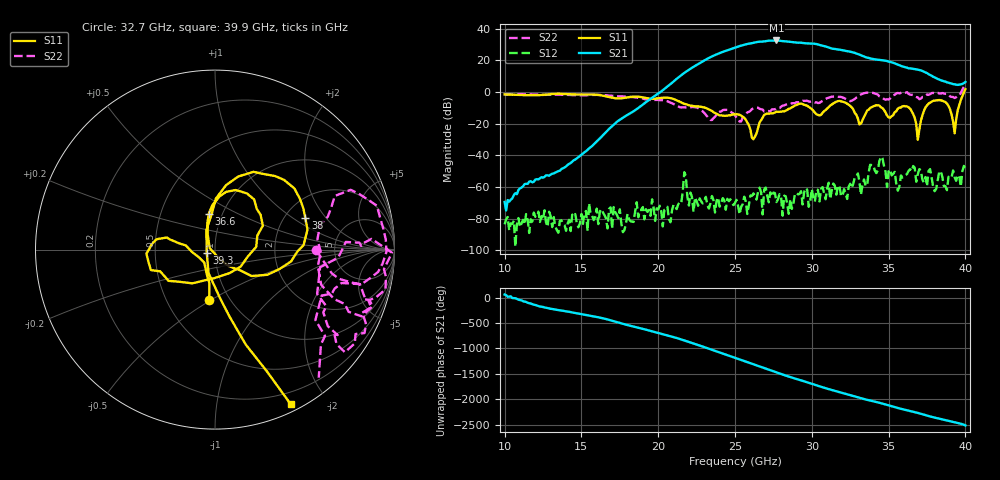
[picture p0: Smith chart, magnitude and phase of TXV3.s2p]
!Keysight Technologies,M9808A,MY58100618,A.14.70.03
!Date: Monday, February 27, 2023 13:37:35
!Correction: S11(C  2-Port  )
!S21(C  2-Port  )
!S12(C  2-Port  )
!S22(C  2-Port  )
!S2P File: Measurements: S11, S21, S12, S22:
# Hz S  RI  R 50
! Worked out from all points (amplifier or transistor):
!   301 points, 10 GHz to 40 GHz, reference 50 ohm
!   highest |S21| = 32.6 dB at 27.7 GHz (marker M1)
!   |S21| within 3 dB of that: 25.49 GHz to 30.57 GHz (5.074 GHz wide, 18.1 % of centre)
!   unconditionally stable (mu >= 1): start of sweep to 33.74 GHz; 34.02 GHz to 39.74 GHz
!   at 15 GHz: K = 40991.98, MAG = -30.4 dB, |S12| = -77.1 dB
!   at 25 GHz: K = 58.31, MAG = 28.4 dB, |S12| = -70.1 dB
!   at 40 GHz: K = 75.33, MSG = 27.2 dB, |S12| = -48.1 dB
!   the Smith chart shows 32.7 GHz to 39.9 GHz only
!   S11 on the Smith chart (normalised r, x): 32.7 GHz: 0.80, -0.49; 36.6 GHz: 0.86, +0.36; 38 GHz: 2.57, +1.28; 39.3 GHz: 0.91, -0.03; 39.9 GHz: 0.07, -1.60
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1e10  0.7154 0.4369  0.000175 0.000287  -4.76e-05 4.53e-05  0.0522 0.8387
1.5e10  0.6422 -0.5324  0.00846 0.00599  -0.000134 4.07e-05  0.7521 0.2094
2e10  -0.207 -0.5991  0.811 0.3794  0.00015 -0.000124  0.2616 -0.498
2.34e10  -0.2586 -0.0696  5.365 11.43  0.00022 -0.000202  -0.0317 -0.1271
2.42e10  -0.1724 0.0531  17.39 -6.275  0.000436 -8.87e-05  -0.2128 -0.1627
2.5e10  -0.1398 0.1381  -5.736 -24.78  0.000313 -1.59e-05  -0.1301 -0.1284
2.59e10  -0.0435 0.079  -31.95 10.84  -0.00011 -0.000234  -0.1949 0.1324
2.66e10  0.1089 -0.0158  2.69 38.5  -0.000915 0.000253  -0.2331 0.1783
2.72e10  0.1827 -0.0976  38.58 16.35  0.000319 7.91e-05  -0.1526 0.1981
2.77e10  0.1876 -0.1482  36.53 -21.81  0.00015 -0.000297  -0.0255 0.3028
2.83e10  0.0906 -0.2398  -1.16 -39.63  -0.000278 -0.000423  0.0366 0.3964
2.9e10  0.0583 -0.3843  -33.75 -13.63  -0.00033 -0.000559  0.0991 0.4645
3e10  0.0898 -0.2728  -10.62 32.31  -0.000862 -2.65e-05  0.2087 0.4649
3.1e10  -0.2538 -0.1589  25.87 5.073  -0.00028 0.000849  0.5658 0.2917
3.19e10  -0.2721 -0.4266  9.468 -19.19  -0.000332 0.000413  0.5678 0.4056
3.27e10  -0.0328 -0.2797  -12.24 -12.87  -0.000522 -0.00113  0.5646 -0.00395
3.5e10  -0.00214 -0.1584  6.533 6.368  0.00237 0.00205  0.573 -0.0928
3.66e10  -0.0347 0.1992  0.8906 -5.306  -0.00364 -0.00281  0.8046 0.0382
3.8e10  0.5029 0.1776  -2.768 0.8086  0.000671 0.000298  0.7829 -0.4705
3.93e10  -0.0458 -0.0191  0.5251 1.672  -0.00172 -0.00102  0.5941 -0.2561
3.99e10  0.4226 -0.8629  1.741 0.7673  -0.0035 0.00302  0.9293 -1.128
4e10  0.5706 -1.088  2.057 0.3411  -0.0032 -0.00233  1.122 -1.502
